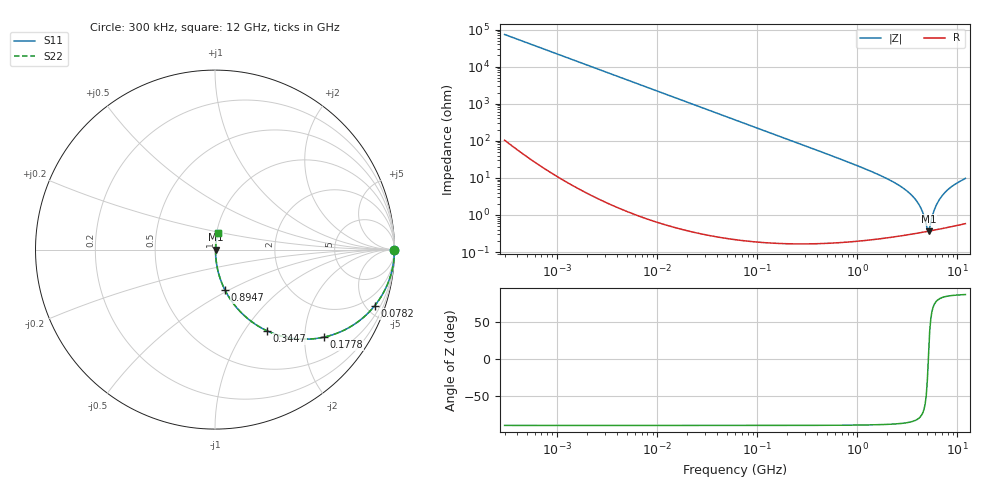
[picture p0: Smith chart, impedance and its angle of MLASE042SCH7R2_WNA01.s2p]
! MLASE042SCH7R2_WNA01  S-PARAMETER MODEL  ( General Type )
! Model Generated by TAIYO YUDEN Corporation (http://www.ty-top.com)
! Version 1.0
! TAIYO YUDEN Control No. 120810
! Copyright(c) 2012 TAIYO YUDEN CO.,LTD. All Rights Reserved.
! Product Description (link to TY-COMPAS)
! https://ds.yuden.co.jp/TYCOMPAS/or/detail?pn=MLASE042SCH7R2BWNA01&u=M
! Products Name : Multilayer Ceramic Capacitors
! Characteristics :
!  Capacitance : 7.2 pF , Rated Voltage : 16V , TCC : CH / C0H
!  Case Size : 0.4 x 0.2 / 0.016 x 0.008 [mm/inch] , Thickness : 0.2 / 0.008 [mm/inch]
!  (Conditions: Temperature = 25 degC , DC Bias Current/Voltage = 0A / 0V)
! External Node Assignments :
!  1  o---| |---o  2
! GND o---------o GND
! Frequency Range : 0.3MHz  -  12000MHz  [ 401 STEP ]
# MHz S RI R 50
! Freq[MHz].  S11 Real  S11 Imag  S21 Real  S21 Imag  S12 Real  S12 Imag  S22 Real  S22 Imag
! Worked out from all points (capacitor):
!   401 points, 300 kHz to 12 GHz, reference 50 ohm
!   read as one part in series: C = 7.2 pF near 316.3 kHz
!   lowest |Z| = 366 mohm at 5.141 GHz (marker M1)
!   series resonance near 5.121 GHz, so ESL is about 130 pH
!   S11 on the Smith chart (normalised r, x): 300 kHz: open; 78.2 MHz: 1.00, -5.66; 177.8 MHz: 1.00, -2.49; 344.7 MHz: 1.00, -1.28; 894.7 MHz: 1.00, -0.48; 12 GHz: 1.01, +0.19
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0.3  1 -0.00136  3.75e-06 0.00136  3.75e-06 0.00136  1 -0.00136
1.769972  0.9999 -0.008  6.69e-05 0.008  6.69e-05 0.008  0.9999 -0.008
10.44266  0.9978 -0.0471  0.00224 0.0471  0.00224 0.0471  0.9978 -0.0471
27.10171  0.9852 -0.1207  0.0148 0.1207  0.0148 0.1207  0.9852 -0.1207
60  0.9313 -0.2526  0.0687 0.2526  0.0687 0.2526  0.9313 -0.2526
78.19928  0.8887 -0.3142  0.1113 0.3142  0.1113 0.3142  0.8887 -0.3142
177.7716  0.6068 -0.4878  0.3932 0.4878  0.3932 0.4878  0.6068 -0.4878
344.7396  0.2902 -0.4526  0.7098 0.4526  0.7098 0.4526  0.2902 -0.4526
353.9943  0.2794 -0.4474  0.7206 0.4474  0.7206 0.4474  0.2794 -0.4474
555.3718  0.1352 -0.3398  0.8648 0.3398  0.8648 0.3398  0.1352 -0.3398
894.6982  0.0559 -0.2258  0.9441 0.2258  0.9441 0.2258  0.0559 -0.2258
2088.533  0.0101 -0.0872  0.9899 0.0872  0.9899 0.0872  0.0101 -0.0872
2947.191  0.0053 -0.0498  0.9947 0.0498  0.9947 0.0498  0.0053 -0.0498
3740.715  0.00387 -0.0274  0.9961 0.0274  0.9961 0.0274  0.00387 -0.0274
4270.516  0.00356 -0.0156  0.9964 0.0156  0.9964 0.0156  0.00356 -0.0156
4875.354  0.00355 -0.00419  0.9964 0.00419  0.9964 0.00419  0.00355 -0.00419
5140.631  0.00363 0.000334  0.9964 -0.000334  0.9964 -0.000334  0.00363 0.000334
5420.343  0.00375 0.00515  0.9962 -0.00515  0.9962 -0.00515  0.00375 0.00515
6026.253  0.00418 0.0156  0.9958 -0.0156  0.9958 -0.0156  0.00418 0.0156
7064.448  0.00537 0.0329  0.9946 -0.0329  0.9946 -0.0329  0.00537 0.0329
8732.115  0.0081 0.0571  0.9919 -0.0571  0.9919 -0.0571  0.0081 0.0571
12000  0.0149 0.095  0.9851 -0.095  0.9851 -0.095  0.0149 0.095
